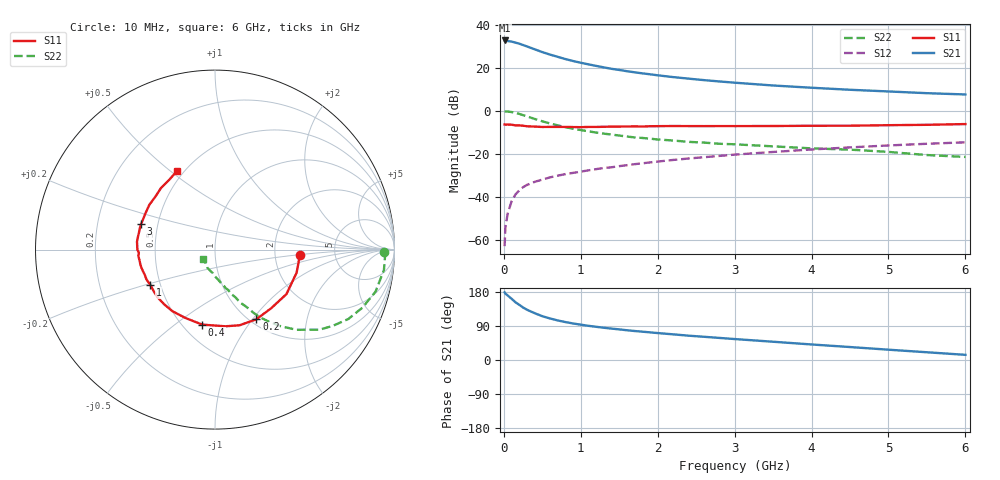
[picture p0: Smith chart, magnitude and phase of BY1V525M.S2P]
! SIEMENS Small Signal Semiconductors
! BFY420
! Si NPN RF SIEGET Grounded Emitter Transistor in MICRO-X
! VCE = 1.5 V  IC = 25 mA
! Common Emitter S-Parameters:  October  1996
# GHz  S  MA  R  50
!  f  S11  S21  S12  S22
! GHz  MAG  ANG  MAG  ANG  MAG  ANG  MAG  ANG
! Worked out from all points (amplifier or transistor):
!   36 points, 10 MHz to 6 GHz, reference 50 ohm
!   highest |S21| = 32.6 dB at 10 MHz (marker M1)
!   |S21| within 3 dB of that: start of sweep to 317 MHz
!   unconditionally stable (mu >= 1): start of sweep to 12.19 MHz; 1.684 GHz to end of sweep
!   at 250 MHz: K = 0.34, MSG = 33.1 dB, |S12| = -35.7 dB
!   at 1.4 GHz: K = 0.96, MSG = 22.9 dB, |S12| = -26.4 dB
!   at 6 GHz: K = 1.08, MAG = 9.4 dB, |S12| = -14.8 dB
!   S11 on the Smith chart (normalised r, x): 10 MHz: 2.79, -0.23; 200 MHz: 1.07, -1.05; 400 MHz: 0.62, -0.63; 1 GHz: 0.44, -0.21; 3 GHz: 0.40, +0.14; 6 GHz: 0.46, +0.53
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0.01  0.4749 -3.8  42.73 178.6  0.0007 101.1  0.9421 -0.7
0.02  0.4716 -6.9  42.67 175.4  0.0019 87.9  0.9482 -2.2
0.1  0.4689 -31.9  40.24 161.8  0.0077 77.5  0.9245 -14.7
0.15  0.4526 -46.0  38.09 152.5  0.0111 72.4  0.8827 -21.5
0.2  0.4515 -59.2  35.99 145.7  0.0139 71.4  0.8373 -27.5
0.25  0.4433 -72.0  33.45 138.5  0.0165 66.3  0.782 -32.9
0.3  0.4312 -82.3  31.04 132.7  0.0186 64.8  0.7342 -37.4
0.4  0.4239 -99.7  26.67 123.6  0.0219 60.6  0.6387 -44.4
0.5  0.415 -113.5  22.88 115.6  0.0248 59.1  0.5628 -49.4
0.6  0.4172 -124.6  20.06 109.6  0.0279 57.6  0.5012 -53.2
0.7  0.4161 -132.7  17.78 104.4  0.0306 58.0  0.4527 -56.4
0.8  0.4158 -140.2  15.77 100.1  0.0332 57.1  0.4111 -58.7
1  0.4105 -151.3  12.94 93.2  0.0379 57.8  0.3521 -62.2
1.1  0.4164 -156.4  11.88 90.2  0.0407 58.4  0.3288 -64.3
1.4  0.4229 -166.9  9.351 82.9  0.0479 58.4  0.2767 -68.2
1.6  0.4252 -172.3  8.229 78.5  0.0536 58.0  0.2487 -71.0
2.2  0.4367 174.2  6.004 67.7  0.0709 55.8  0.2011 -77.7
3  0.4352 161.1  4.451 55.3  0.0943 51.4  0.1641 -85.4
3.5  0.4368 152.9  3.828 48.2  0.1088 47.7  0.1469 -90.7
4.5  0.4443 138.4  3.044 34.2  0.1391 39.0  0.1232 -101.2
5.5  0.466 122.9  2.536 20.4  0.1688 29.4  0.0922 -123.7
6  0.485 116.0  2.368 13.6  0.1824 24.3  0.0833 -142.1
